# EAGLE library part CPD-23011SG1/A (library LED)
CPD23011 7-segment LED
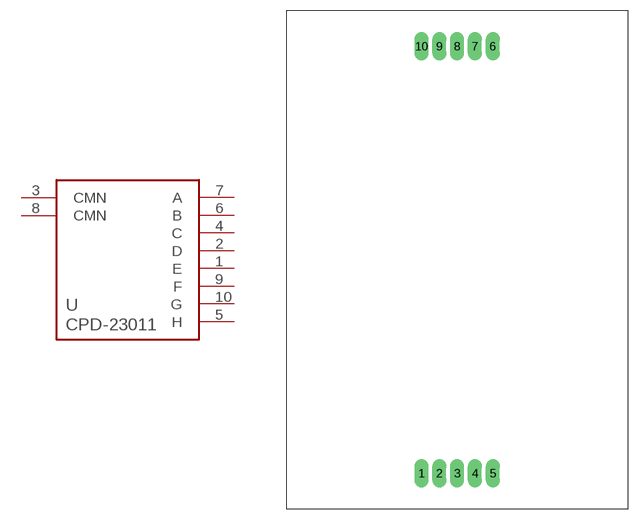
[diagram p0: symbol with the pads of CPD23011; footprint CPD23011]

Designator prefix -

## CPD-23011SG1/A  [CPD23011]
1  E
2  D
3  CMN
4  C
5  H
6  B
7  A
8  CMN
9  F
10  G

## Footprint CPD23011 (pad centres in mm)
drill 0.5 pad 2 long: 1 -5,-30; 2 -2.5,-30; 3 0,-30; 4 2.5,-30; 5 5,-30; 6 5,30; 7 2.5,30; 8 0,30; 9 -2.5,30; 10 -5,30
